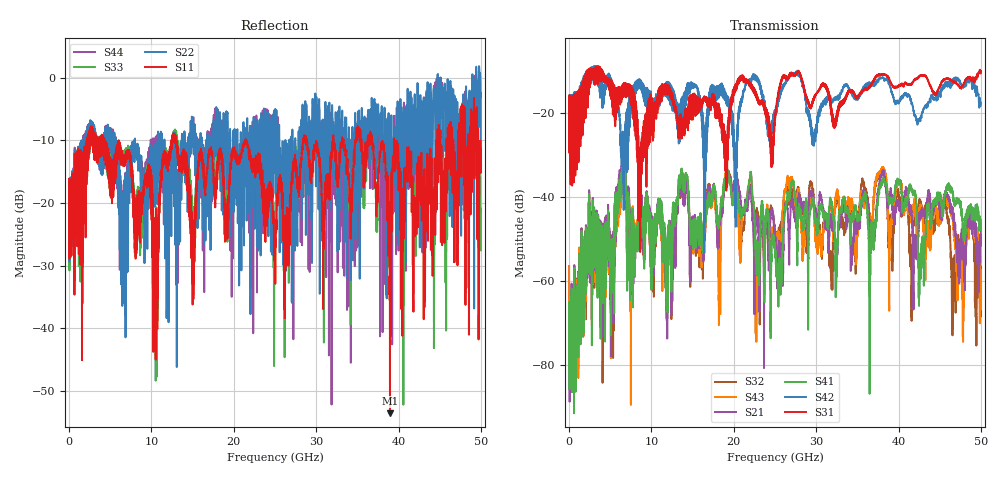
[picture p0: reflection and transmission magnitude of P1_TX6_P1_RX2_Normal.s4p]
!Keysight Technologies,N5225B,MY57041031,A.13.20.10
!Date: Friday, May 31, 2019 11:15:57
!Correction: S11(Full 4 Port(1,2,3,4))
!S12(Full 4 Port(1,2,3,4))
!S13(Full 4 Port(1,2,3,4))
!S14(Full 4 Port(1,2,3,4))
!S21(Full 4 Port(1,2,3,4))
!S22(Full 4 Port(1,2,3,4))
!S23(Full 4 Port(1,2,3,4))
!S24(Full 4 Port(1,2,3,4))
!S31(Full 4 Port(1,2,3,4))
!S32(Full 4 Port(1,2,3,4))
!S33(Full 4 Port(1,2,3,4))
!S34(Full 4 Port(1,2,3,4))
!S41(Full 4 Port(1,2,3,4))
!S42(Full 4 Port(1,2,3,4))
!S43(Full 4 Port(1,2,3,4))
!S44(Full 4 Port(1,2,3,4))
!S4P File: Measurements: <S11,S12,S13,S14>,
!<S21,S22,S23,S24>,
!<S31,S32,S33,S34>,
!<S41,S42,S43,S44>:
# Hz S  dB  R 50.0
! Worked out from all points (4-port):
!   5000 points, 10 MHz to 50 GHz, reference 50 ohm
!   strongest paths, dB at 10 MHz, 12.51 GHz, 25.01 GHz, 37.51 GHz, 50 GHz:
!     S31: -19.4, -15.5, -21.6, -10.8, -9.9
!     S42: -19.4, -16.3, -19.6, -12.3, -17.4
!     S41: -70.3, -46.8, -54.1, -41.1, -45.3
!     S21: -65.3, -51.5, -49.6, -38.8, -46.8
!     S43: -56.4, -46.4, -50.6, -34.7, -66.6
!     S32: -66.2, -51.4, -48.3, -35.7, -58.7
!   lowest |S11| = -53.6 dB at 38.96 GHz (marker M1), VSWR 1.00, Z = 50.2 + j0.142 ohm
!   |S11| at or under -10 dB: 4.286 GHz to 12.47 GHz (8.179 GHz wide, 97.7 % of centre); 13.02 GHz to 21.43 GHz (8.403 GHz wide, 48.8 % of centre); 21.46 GHz to 28.42 GHz (6.96 GHz wide, 27.9 % of centre)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
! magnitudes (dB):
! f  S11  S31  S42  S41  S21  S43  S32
! 10 MHz  -19.4  -19.4  -19.4  -70.3  -65.3  -56.4  -66.2
! 6.62 GHz  -13.0  -12.9  -28.4  -32.5  -31.4  -33.3  -32.0
! 8.62 GHz  -21.0  -36.1  -13.5  -42.4  -40.4  -42.2  -39.9
! 25.54 GHz  -17.7  -13.7  -16.3  -56.2  -51.2  -49.5  -48.3
! 27.08 GHz  -16.1  -10.4  -10.7  -36.1  -40.7  -35.7  -38.6
! 38.96 GHz  -53.6  -12.3  -13.5  -40.5  -39.1  -52.1  -44.8
! 50 GHz  -11.4  -9.9  -17.4  -45.3  -46.8  -66.6  -58.7
